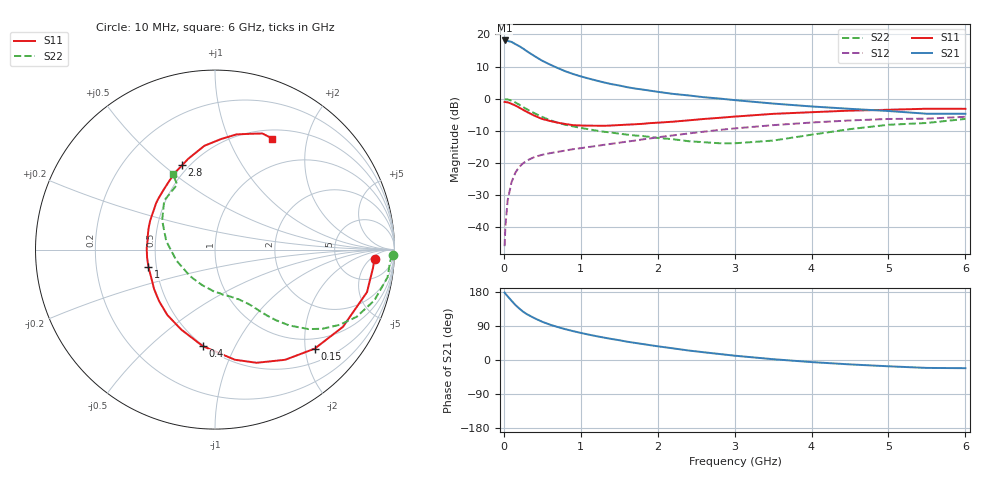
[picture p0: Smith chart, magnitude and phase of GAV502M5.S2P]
! Infineon Technologies  Discrete & RF Semiconductors
! BF775
! Si NPN RF Bipolar Junction Transistor in SOT23
! VCE = 0.5 V  IC = 2.5 mA
! Common Emitter S-Parameters:  May  1996
# GHz  S  MA  R  50
!  f  S11  S21  S12  S22
! GHz  MAG  ANG  MAG  ANG  MAG  ANG  MAG  ANG
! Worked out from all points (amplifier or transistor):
!   36 points, 10 MHz to 6 GHz, reference 50 ohm
!   highest |S21| = 18.1 dB at 10 MHz (marker M1)
!   |S21| within 3 dB of that: start of sweep to 278.9 MHz
!   unconditionally stable (mu >= 1): 904.7 MHz to end of sweep
!   at 250 MHz: K = 0.36, MSG = 17.8 dB, |S12| = -20.1 dB
!   at 1.4 GHz: K = 1.21, MAG = 6.5 dB, |S12| = -14.0 dB
!   at 6 GHz: K = 1.09, MAG = -1.4 dB, |S12| = -5.6 dB
!   S11 on the Smith chart (normalised r, x): 10 MHz: 14, -7; 150 MHz: 0.77, -2.20; 400 MHz: 0.49, -0.75; 1 GHz: 0.45, -0.10; 2.8 GHz: 0.46, +0.58; 6 GHz: 0.61, +1.46
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0.01  0.8903 -3.2  8.047 177.9  0.0051 88.6  0.9905 -1.8
0.02  0.8864 -6.5  7.977 175.0  0.0103 88.1  0.9781 -3.7
0.05  0.8794 -15.6  7.897 168.0  0.0265 80.6  0.9736 -9.1
0.1  0.8327 -31.1  7.647 156.4  0.0504 72.3  0.9318 -17.7
0.15  0.783 -44.8  7.062 145.2  0.0709 64.2  0.8734 -25.4
0.2  0.7279 -57.5  6.558 136.0  0.0869 58.8  0.81 -31.2
0.25  0.6719 -69.8  6.026 127.6  0.099 53.5  0.7431 -36.4
0.3  0.6236 -79.8  5.468 120.9  0.1093 49.8  0.6849 -40.3
0.4  0.5421 -97.2  4.586 110.2  0.1243 44.6  0.5933 -45.5
0.5  0.4837 -112.9  3.883 100.8  0.1345 41.2  0.5199 -49.2
0.6  0.4508 -126.1  3.399 93.3  0.1423 39.5  0.4645 -51.9
0.7  0.4239 -137.3  2.999 87.0  0.1491 38.7  0.4242 -53.9
0.8  0.4042 -147.1  2.669 81.3  0.1564 38.0  0.3937 -55.6
1  0.3834 -165.2  2.225 71.5  0.1703 37.7  0.3521 -58.7
1.1  0.381 -173.3  2.063 67.1  0.1773 37.7  0.3353 -60.7
1.6  0.3951 156.3  1.513 48.4  0.2153 38.1  0.2766 -71.5
2.2  0.4394 130.7  1.188 30.7  0.269 36.2  0.2346 -90.9
2.8  0.5042 111.3  1.007 15.9  0.327 31.7  0.2032 -121.2
3.5  0.5815 95.8  0.841 2.1  0.388 23.9  0.2234 -164.1
4.5  0.6531 79.4  0.696 -11.6  0.4593 11.6  0.3366 151.0
5.5  0.6988 67.8  0.584 -20.9  0.4897 -1.4  0.4197 120.1
6  0.6963 62.7  0.583 -21.6  0.5236 -4.9  0.4853 119.2
